(* Logix 5000 Controller export Example_PLC; controller Example_PLC 1769-L32E rev 19.11; software revision 19.01; part 4 of 6 *)
(* tags used below, declared in another part *)
   Mode_Requested : SINT;   // Drive Mode Requested (0=Position, 1=Velocity, 2=Torque)
   Mode_Actual : SINT;   // Drive Mode Actual (0=Position, 1=Velocity, 2=Torque)
   ErrorSource : SINT;   // Source of Error
   Get_Mode : AKD_Get_Attribute;
   Set_Mode : AKD_Set_Attribute;
(* AKD_Set_Mode, continued *)

ROUTINE Logic   (* ladder *)
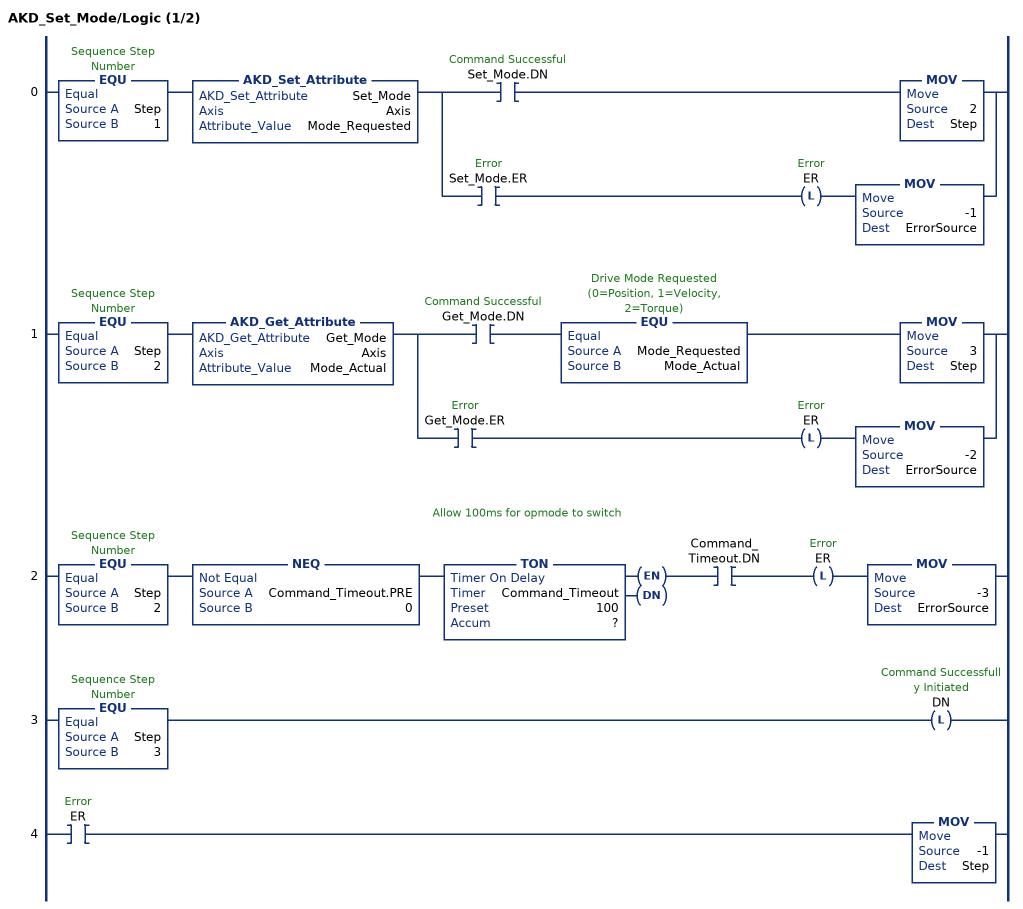
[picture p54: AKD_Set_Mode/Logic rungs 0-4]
   0: EQU(Step,1)AKD_Set_Attribute(Set_Mode,Axis,Mode_Requested)[XIC(Set_Mode.DN) MOV(2,Step) ,XIC(Set_Mode.ER) OTL(ER) MOV(-1,ErrorSource) ];
   1: EQU(Step,2)AKD_Get_Attribute(Get_Mode,Axis,Mode_Actual)[XIC(Get_Mode.DN) EQU(Mode_Requested,Mode_Actual) MOV(3,Step) ,XIC(Get_Mode.ER) OTL(ER) MOV(-2,ErrorSource) ];
   // Allow 100ms for opmode to switch
   2: EQU(Step,2)NEQ(Command_Timeout.PRE,0)TON(Command_Timeout,?,?)XIC(Command_Timeout.DN)OTL(ER)MOV(-3,ErrorSource);
   3: EQU(Step,3)OTL(DN);
   4: XIC(ER)MOV(-1,Step);
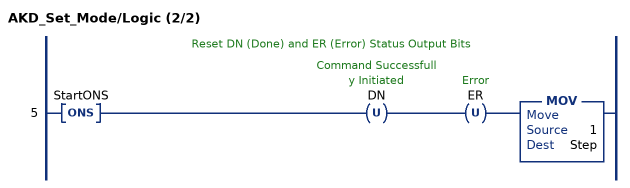
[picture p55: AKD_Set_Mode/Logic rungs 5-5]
   // Reset DN (Done) and ER (Error) Status Output Bits
   5: ONS(StartONS)OTU(DN)OTU(ER)MOV(1,Step);
END_ROUTINE

ROUTINE Prescan   (* ladder *)
// Prescan
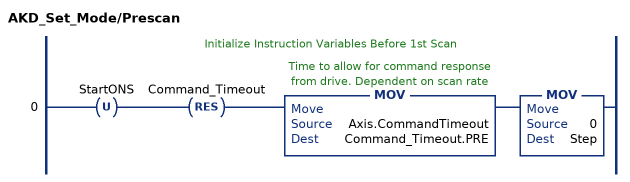
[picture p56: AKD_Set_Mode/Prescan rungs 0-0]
   // Initialize Instruction Variables Before 1st Scan
   0: OTU(StartONS)RES(Command_Timeout)MOV(Axis.CommandTimeout,Command_Timeout.PRE)MOV(0,Step);
END_ROUTINE
END_ADD_ON_INSTRUCTION

ADD_ON_INSTRUCTION AKD_Get_Parameter   (* revision 2.0, ExecutePrescan, ExecuteEnableInFalse *)
// Get Drive Parameter
VAR_OUTPUT
   DN : BOOL; {access Read Only, visible}   // Command Successful
   ER : BOOL; {access Read Only, visible}   // Error
END_VAR
VAR_IN_OUT
   Axis : AKD_Axis; {required}
END_VAR
VAR_INPUT
   Parameter_Number : INT; {visible}   // See help (F1) for parameter list.
END_VAR
VAR_OUTPUT
   Parameter_Value : DINT; {access Read Only, required}   // Parameter Value
END_VAR
VAR
   Command_Timeout : TIMER := (PRE := 2000);   // Timeout Timer
   Command_Message_Type : SINT;   // Command Message Type
   Command_Axis_Number : SINT;   // Command Axis Number
   Step : SINT;
   Command_Bytes : SINT[8];
   OS_LoadStart : BOOL;
   Temp_Bytes : SINT[2];   // Temporary Bytes to Split into Command Bytes
END_VAR

ROUTINE EnableInFalse   (* ladder *)
// EnableIn_False
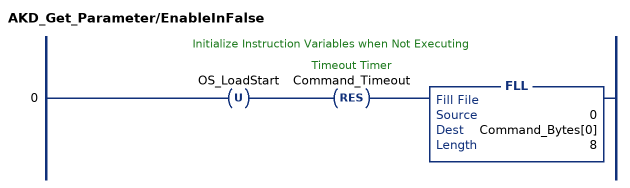
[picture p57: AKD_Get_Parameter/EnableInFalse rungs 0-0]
   // Initialize Instruction Variables when Not Executing
   0: OTU(OS_LoadStart)RES(Command_Timeout)FLL(0,Command_Bytes[0],8);
END_ROUTINE

ROUTINE Logic   (* ladder *)
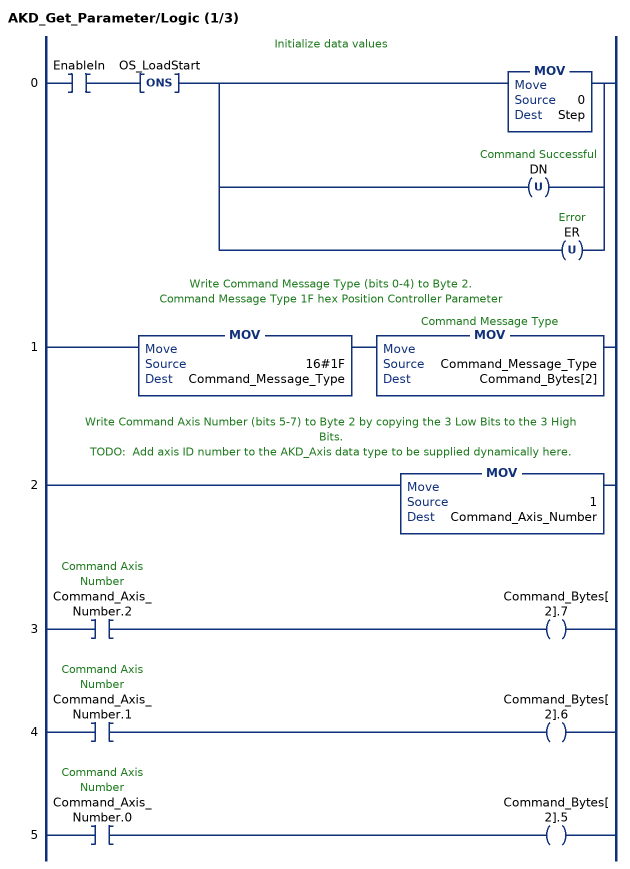
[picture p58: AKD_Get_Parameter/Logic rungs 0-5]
   // Initialize data values
   0: XIC(EnableIn)ONS(OS_LoadStart)[MOV(0,Step) ,OTU(DN) ,OTU(ER) ];
   // Write Command Message Type (bits 0-4) to Byte 2.
   // Command Message Type 1F hex Position Controller Parameter
   1: MOV(16#1F,Command_Message_Type)MOV(Command_Message_Type,Command_Bytes[2]);
   // Write Command Axis Number (bits 5-7) to Byte 2 by copying the 3 Low Bits to the 3 High Bits.
   // TODO:  Add axis ID number to the AKD_Axis data type to be supplied dynamically here.
   2: MOV(1,Command_Axis_Number);
   3: XIC(Command_Axis_Number.2)OTE(Command_Bytes[2].7);
   4: XIC(Command_Axis_Number.1)OTE(Command_Bytes[2].6);
   5: XIC(Command_Axis_Number.0)OTE(Command_Bytes[2].5);
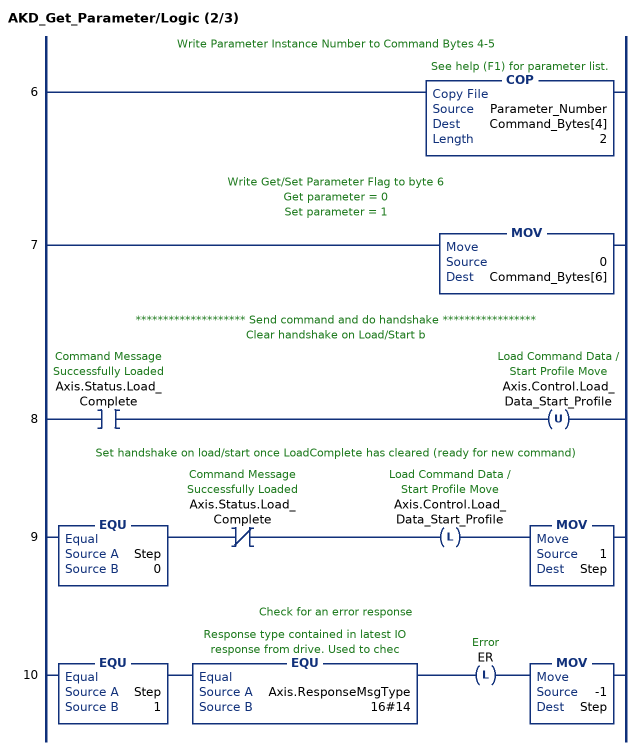
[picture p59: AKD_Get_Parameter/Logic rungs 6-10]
   // Write Parameter Instance Number to Command Bytes 4-5
   6: COP(Parameter_Number,Command_Bytes[4],2);
   // Write Get/Set Parameter Flag to byte 6
   // Get parameter = 0
   // Set parameter = 1
   7: MOV(0,Command_Bytes[6]);
   // ******************** Send command and do handshake *****************
   // Clear handshake on Load/Start b
   8: XIC(Axis.Status.Load_Complete)OTU(Axis.Control.Load_Data_Start_Profile);
   // Set handshake on load/start once LoadComplete has cleared (ready for new command)
   9: EQU(Step,0)XIO(Axis.Status.Load_Complete)OTL(Axis.Control.Load_Data_Start_Profile)MOV(1,Step);
   // Check for an error response
   10: EQU(Step,1)EQU(Axis.ResponseMsgType,16#14)OTL(ER)MOV(-1,Step);
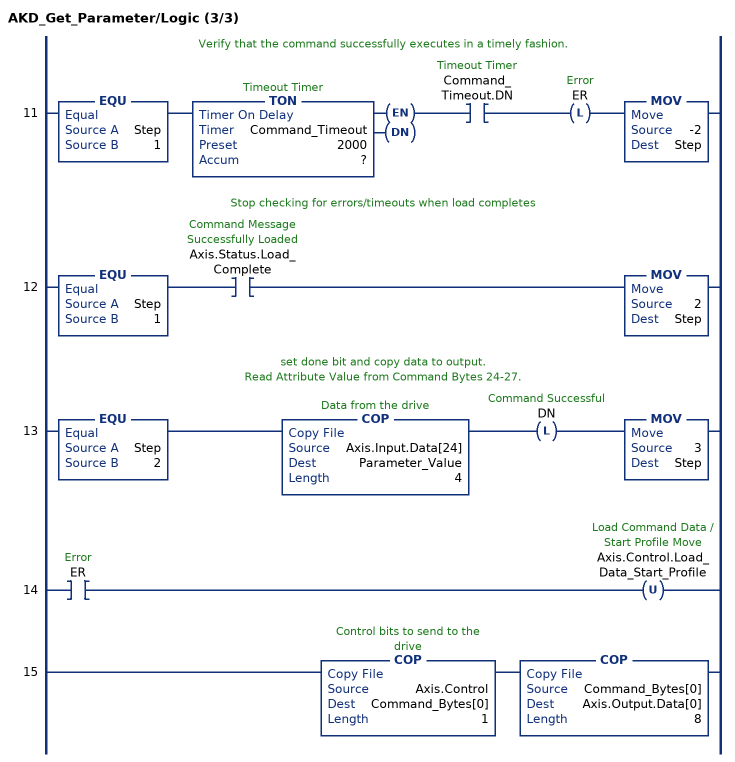
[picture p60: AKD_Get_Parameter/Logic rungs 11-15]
   // Verify that the command successfully executes in a timely fashion.
   11: EQU(Step,1)TON(Command_Timeout,?,?)XIC(Command_Timeout.DN)OTL(ER)MOV(-2,Step);
   // Stop checking for errors/timeouts when load completes
   12: EQU(Step,1)XIC(Axis.Status.Load_Complete)MOV(2,Step);
   // set done bit and copy data to output.
   // Read Attribute Value from Command Bytes 24-27.
   13: EQU(Step,2)COP(Axis.Input.Data[24],Parameter_Value,4)OTL(DN)MOV(3,Step);
   14: XIC(ER)OTU(Axis.Control.Load_Data_Start_Profile);
   15: COP(Axis.Control,Command_Bytes[0],1)COP(Command_Bytes[0],Axis.Output.Data[0],8);
END_ROUTINE

ROUTINE Prescan   (* ladder *)
// Prescan
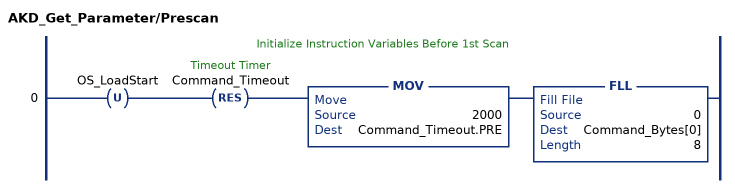
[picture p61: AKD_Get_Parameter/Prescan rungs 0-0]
   // Initialize Instruction Variables Before 1st Scan
   0: OTU(OS_LoadStart)RES(Command_Timeout)MOV(2000,Command_Timeout.PRE)FLL(0,Command_Bytes[0],8);
END_ROUTINE
END_ADD_ON_INSTRUCTION

ADD_ON_INSTRUCTION AKD_Home   (* revision 2.1, ExecutePrescan, ExecuteEnableInFalse *)
// Home Axis
// Revision note:
// IP ouput bit should be turned off when the enable input is false
VAR_OUTPUT
   DN : BOOL; {access Read Only, visible}   // Command Successfully Initiated
   ER : BOOL; {access Read Only, visible}   // Error
   IP : BOOL; {access Read Only, visible}   // Command in Process
   PC : BOOL; {access Read Only, visible}   // Command Process Complete
END_VAR
VAR_IN_OUT
   Axis : AKD_Axis; {required}
END_VAR
VAR
   Step : SINT;
   Set_Attribute : AKD_Set_Attribute;
   Value : DINT;
   StartONS : BOOL;
END_VAR

ROUTINE EnableInFalse   (* ladder *)
// EnableIn_False
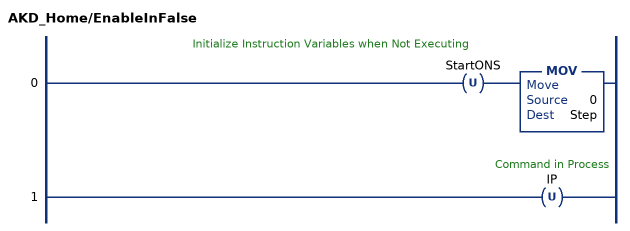
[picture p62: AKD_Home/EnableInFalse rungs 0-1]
   // Initialize Instruction Variables when Not Executing
   0: OTU(StartONS)MOV(0,Step);
   1: OTU(IP);
END_ROUTINE

ROUTINE Logic   (* ladder *)
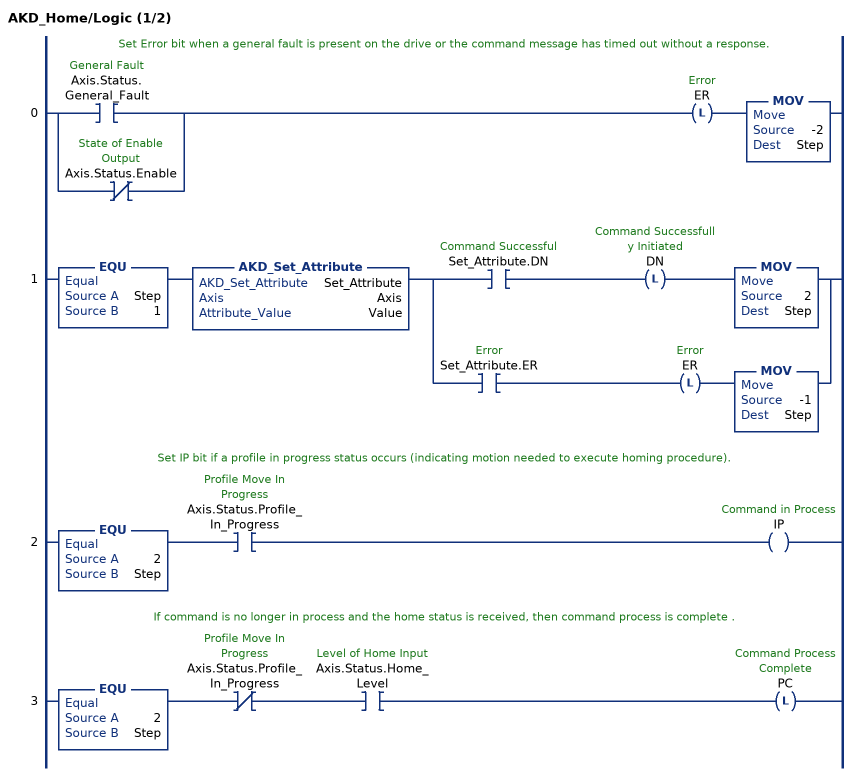
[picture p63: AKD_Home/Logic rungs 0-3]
   // Set Error bit when a general fault is present on the drive or the command message has timed out without a response.
   0: [XIC(Axis.Status.General_Fault) ,XIO(Axis.Status.Enable) ]OTL(ER)MOV(-2,Step);
   1: EQU(Step,1)AKD_Set_Attribute(Set_Attribute,Axis,Value)[XIC(Set_Attribute.DN) OTL(DN) MOV(2,Step) ,XIC(Set_Attribute.ER) OTL(ER) MOV(-1,Step) ];
   // Set IP bit if a profile in progress status occurs (indicating motion needed to execute homing procedure).
   2: EQU(2,Step)XIC(Axis.Status.Profile_In_Progress)OTE(IP);
   // If command is no longer in process and the home status is received, then command process is complete .
   3: EQU(2,Step)XIO(Axis.Status.Profile_In_Progress)XIC(Axis.Status.Home_Level)OTL(PC);
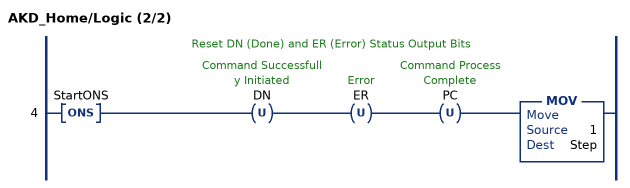
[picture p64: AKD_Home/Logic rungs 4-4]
   // Reset DN (Done) and ER (Error) Status Output Bits
   4: ONS(StartONS)OTU(DN)OTU(ER)OTU(PC)MOV(1,Step);
END_ROUTINE

ROUTINE Prescan   (* ladder *)
// Prescan
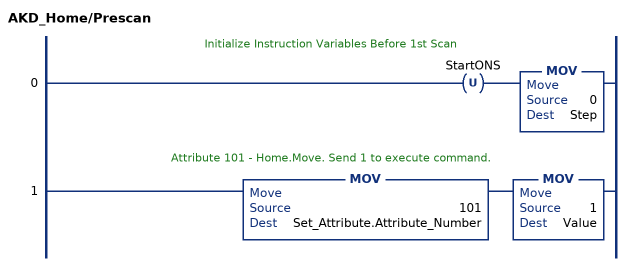
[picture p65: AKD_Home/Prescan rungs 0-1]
   // Initialize Instruction Variables Before 1st Scan
   0: OTU(StartONS)MOV(0,Step);
   // Attribute 101 - Home.Move. Send 1 to execute command.
   1: MOV(101,Set_Attribute.Attribute_Number)MOV(1,Value);
END_ROUTINE
END_ADD_ON_INSTRUCTION

ADD_ON_INSTRUCTION AKD_Set_Position   (* revision 2.1, ExecutePrescan, ExecuteEnableInFalse *)
// Set Drive Position
// Revision note:
// Don't error if Command_Timeout preset is 0
VAR_OUTPUT
   DN : BOOL; {access Read Only, visible}   // Command Successful
   ER : BOOL; {access Read Only, visible}   // Error
END_VAR
VAR_IN_OUT
   Axis : AKD_Axis; {required}
END_VAR
VAR_INPUT
   Incremental : BOOL; {visible}   // Position Definition (0=Absolute, 1=Incremental)
   Position : DINT; {required}   // Position Value
END_VAR
VAR_OUTPUT
   PC : BOOL; {access Read Only, visible}   // Process Complete
   IP : BOOL; {access Read Only, visible}   // In Process
END_VAR
VAR
   Response_Bytes : SINT[8];
   OS_LoadStart : BOOL;
   Position_Internal : DINT;   // Scaled Position Value for Drive
   Command_Timeout : TIMER := (PRE := 200);   // Timeout Timer
   Command_Message_Type : SINT;   // Command Message Type
   Command_Axis_Number : SINT;   // Command Axis Number
   Response_Message_Type : SINT;   // Response Message Type
   Response_Axis_Number : SINT;   // Response Axis Number
   Command_Bytes : SINT[8];
   Step : SINT;
END_VAR

ROUTINE EnableInFalse   (* ladder *)
// EnableIn_False
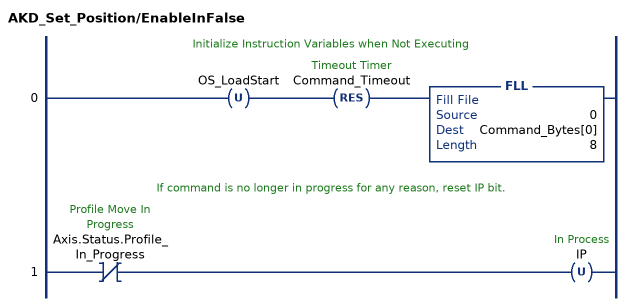
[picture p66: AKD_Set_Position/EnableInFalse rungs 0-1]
   // Initialize Instruction Variables when Not Executing
   0: OTU(OS_LoadStart)RES(Command_Timeout)FLL(0,Command_Bytes[0],8);
   // If command is no longer in progress for any reason, reset IP bit.
   1: XIO(Axis.Status.Profile_In_Progress)OTU(IP);
END_ROUTINE

ROUTINE Logic   (* ladder *)
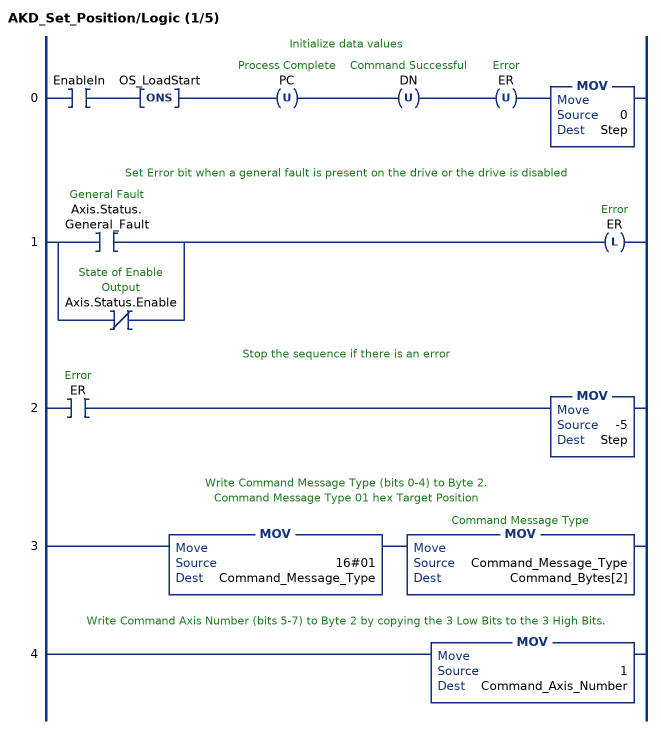
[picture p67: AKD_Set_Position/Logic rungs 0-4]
   // Initialize data values
   0: XIC(EnableIn)ONS(OS_LoadStart)OTU(PC)OTU(DN)OTU(ER)MOV(0,Step);
   // Set Error bit when a general fault is present on the drive or the drive is disabled
   1: [XIC(Axis.Status.General_Fault) ,XIO(Axis.Status.Enable) ]OTL(ER);
   // Stop the sequence if there is an error
   2: XIC(ER)MOV(-5,Step);
   // Write Command Message Type (bits 0-4) to Byte 2.
   // Command Message Type 01 hex Target Position
   3: MOV(16#01,Command_Message_Type)MOV(Command_Message_Type,Command_Bytes[2]);
   // Write Command Axis Number (bits 5-7) to Byte 2 by copying the 3 Low Bits to the 3 High Bits.
   4: MOV(1,Command_Axis_Number);
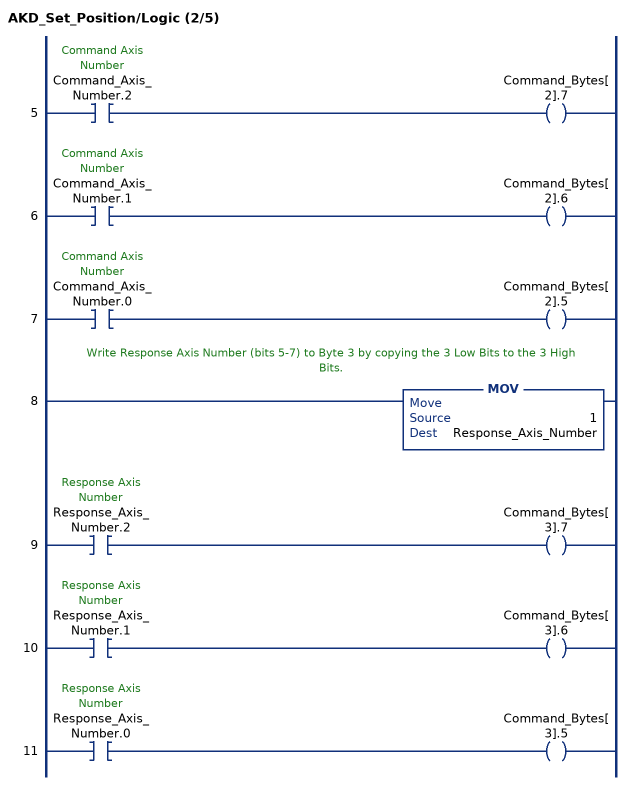
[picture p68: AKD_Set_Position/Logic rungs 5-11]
   5: XIC(Command_Axis_Number.2)OTE(Command_Bytes[2].7);
   6: XIC(Command_Axis_Number.1)OTE(Command_Bytes[2].6);
   7: XIC(Command_Axis_Number.0)OTE(Command_Bytes[2].5);
   // Write Response Axis Number (bits 5-7) to Byte 3 by copying the 3 Low Bits to the 3 High Bits.
   8: MOV(1,Response_Axis_Number);
   9: XIC(Response_Axis_Number.2)OTE(Command_Bytes[3].7);
   10: XIC(Response_Axis_Number.1)OTE(Command_Bytes[3].6);
   11: XIC(Response_Axis_Number.0)OTE(Command_Bytes[3].5);
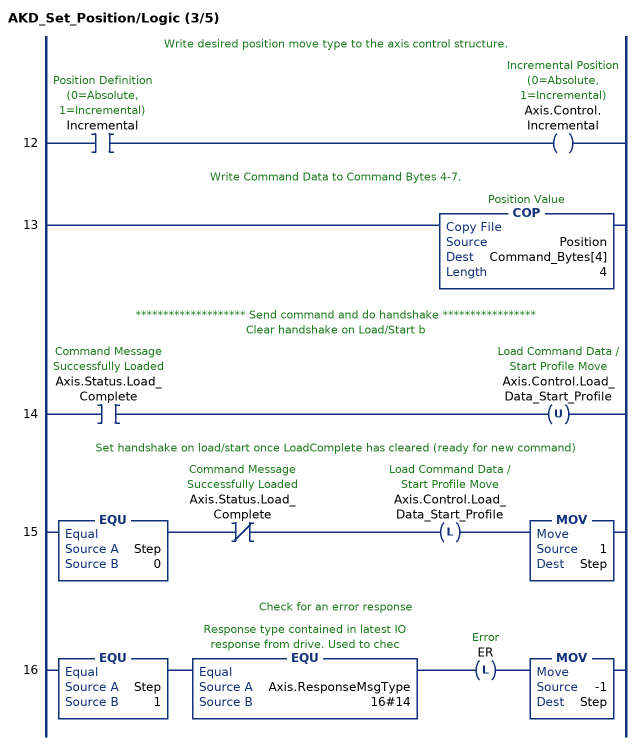
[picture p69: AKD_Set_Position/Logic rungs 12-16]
   // Write desired position move type to the axis control structure.
   12: XIC(Incremental)OTE(Axis.Control.Incremental);
   // Write Command Data to Command Bytes 4-7.
   13: COP(Position,Command_Bytes[4],4);
   // ******************** Send command and do handshake *****************
   // Clear handshake on Load/Start b
   14: XIC(Axis.Status.Load_Complete)OTU(Axis.Control.Load_Data_Start_Profile);
   // Set handshake on load/start once LoadComplete has cleared (ready for new command)
   15: EQU(Step,0)XIO(Axis.Status.Load_Complete)OTL(Axis.Control.Load_Data_Start_Profile)MOV(1,Step);
   // Check for an error response
   16: EQU(Step,1)EQU(Axis.ResponseMsgType,16#14)OTL(ER)MOV(-1,Step);
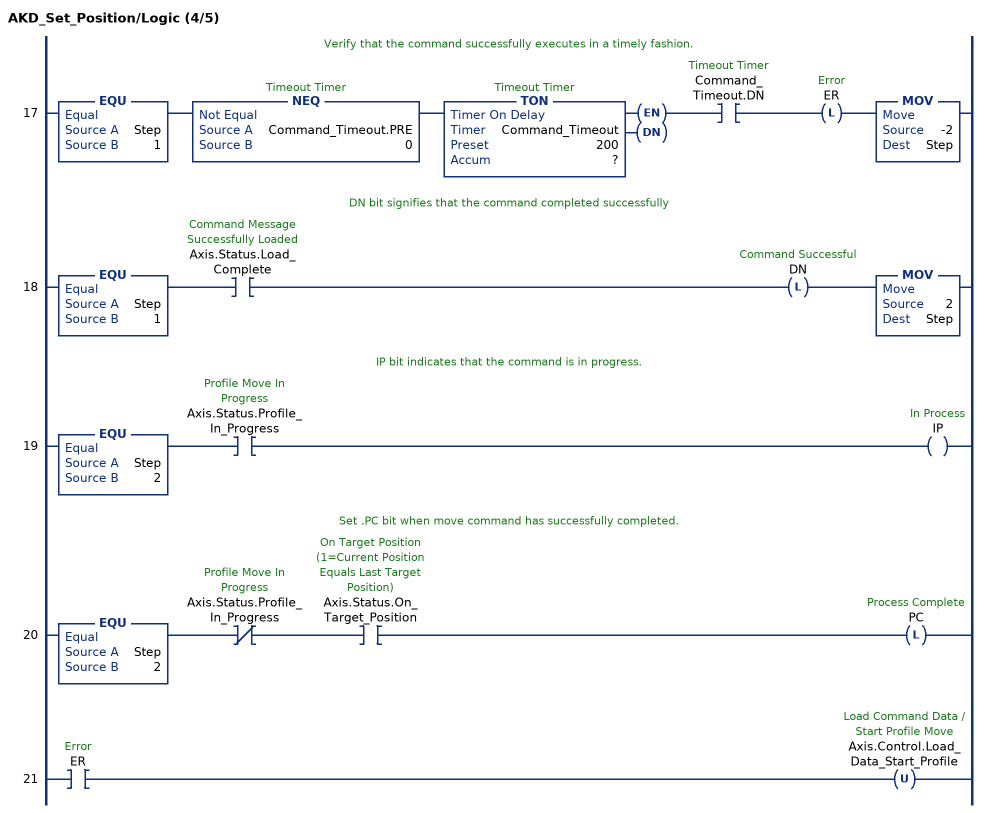
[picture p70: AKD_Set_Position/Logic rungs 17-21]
   // Verify that the command successfully executes in a timely fashion.
   17: EQU(Step,1)NEQ(Command_Timeout.PRE,0)TON(Command_Timeout,?,?)XIC(Command_Timeout.DN)OTL(ER)MOV(-2,Step);
   // DN bit signifies that the command completed successfully
   18: EQU(Step,1)XIC(Axis.Status.Load_Complete)OTL(DN)MOV(2,Step);
   // IP bit indicates that the command is in progress.
   19: EQU(Step,2)XIC(Axis.Status.Profile_In_Progress)OTE(IP);
   // Set .PC bit when move command has successfully completed.
   20: EQU(Step,2)XIO(Axis.Status.Profile_In_Progress)XIC(Axis.Status.On_Target_Position)OTL(PC);
   21: XIC(ER)OTU(Axis.Control.Load_Data_Start_Profile);
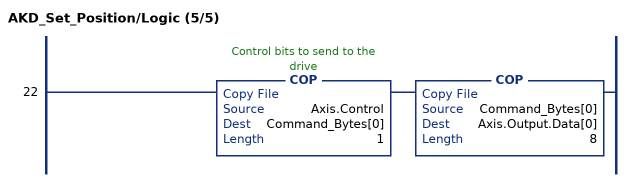
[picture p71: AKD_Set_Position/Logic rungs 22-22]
   22: COP(Axis.Control,Command_Bytes[0],1)COP(Command_Bytes[0],Axis.Output.Data[0],8);
END_ROUTINE
